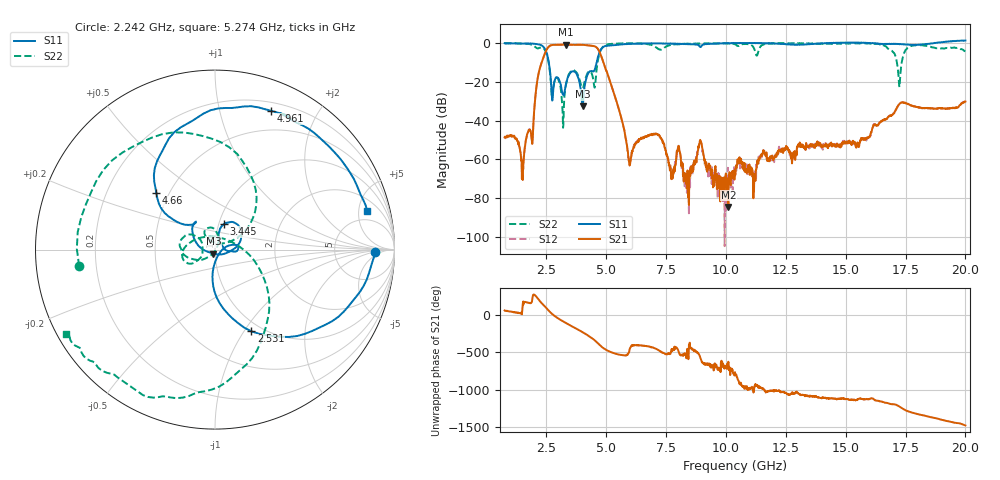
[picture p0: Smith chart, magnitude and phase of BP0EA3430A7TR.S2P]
! s2p File.  Ports: 1,3
# MHz S DB R 50
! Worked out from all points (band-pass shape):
!   1601 points, 750 MHz to 20 GHz, reference 50 ohm
!   highest |S21| = -0.87 dB at 3.301 GHz (marker M1); lowest = -84.5 dB at 10.1 GHz (marker M2)
!   |S21| within 3 dB of the highest: 2.489 GHz to 4.686 GHz (2.197 GHz wide, 61.2 % of centre)
!   lowest |S11| = -32.5 dB at 4.01 GHz (marker M3), VSWR 1.05, Z = 49.1 - j2.16 ohm
!   |S11| at or under -10 dB: 2.596 GHz to 4.597 GHz (2 GHz wide, 55.6 % of centre)
!   |S22| runs from -43.7 to 0.0 dB; largest |S21 - S12| = 0.0096
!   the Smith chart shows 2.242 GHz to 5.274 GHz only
!   S11 on the Smith chart (normalised r, x): 2.242 GHz: 17, -2; 2.531 GHz: 0.89, -1.08; 3.445 GHz: 1.06, +0.31; 4.66 GHz: 0.43, +0.34; 4.961 GHz: 0.29, +1.44; 5.274 GHz: 3.42, +6.25
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750  -0.16 136.4  -48.66 59.9  -49.29 55.8  -0.19 160.5
1520  -0.29 79.0  -64.93 177.9  -64.31 164.2  -0.32 119.0
1989.22  -0.41 32.6  -34.10 -90.1  -34.15 -89.9  -1.62 14.3
2241.88  -0.98 -0.8  -12.17 176.7  -12.20 176.3  -2.36 -173.1
2530.63  -6.06 -66.1  -2.90 79.2  -2.93 79.0  -6.71 64.6
3300.63  -21.92 76.5  -0.87 -106.9  -0.89 -107.3  -22.28 -138.2
3445  -16.35 70.5  -0.94 -132.6  -0.95 -133.0  -15.86 -165.1
3962.34  -27.82 -41.9  -0.94 137.6  -0.95 137.4  -22.65 162.1
4010.47  -32.54 -111.1  -0.96 128.6  -0.98 128.5  -23.19 -175.9
4660.16  -6.87 136.1  -3.33 -24.3  -3.34 -24.5  -8.16 -40.1
4960.94  -1.59 68.0  -13.10 -100.5  -13.13 -100.9  -1.11 -111.0
5273.75  -1.15 14.1  -24.26 -147.6  -24.30 -147.9  -0.40 -150.4
5959.53  -0.50 -61.7  -62.73 -117.7  -62.37 -128.5  -0.27 -176.1
7174.69  -0.22 -99.9  -47.25 -111.2  -47.08 -112.5  -3.12 60.9
7704.06  -0.42 -115.3  -68.20 -135.3  -69.49 -141.4  -0.91 -100.2
10098.28  -0.11 119.3  -84.52 93.7  -67.07 6.7  -0.21 148.0
10375  -0.02 118.6  -65.48 -45.4  -68.12 -51.8  -0.72 139.9
13587.34  -0.51 8.5  -52.95 -2.8  -53.33 -7.5  -0.26 134.4
16799.69  -0.55 20.4  -37.95 -102.3  -37.85 -104.3  -3.31 58.7
17557.66  -0.84 -10.1  -31.16 156.7  -31.23 157.4  -2.83 129.2
18965.31  0.27 -93.1  -33.75 41.6  -33.53 41.8  -2.92 -7.1
20000  1.27 -98.4  -30.17 -37.9  -30.12 -38.0  -4.31 -141.2
